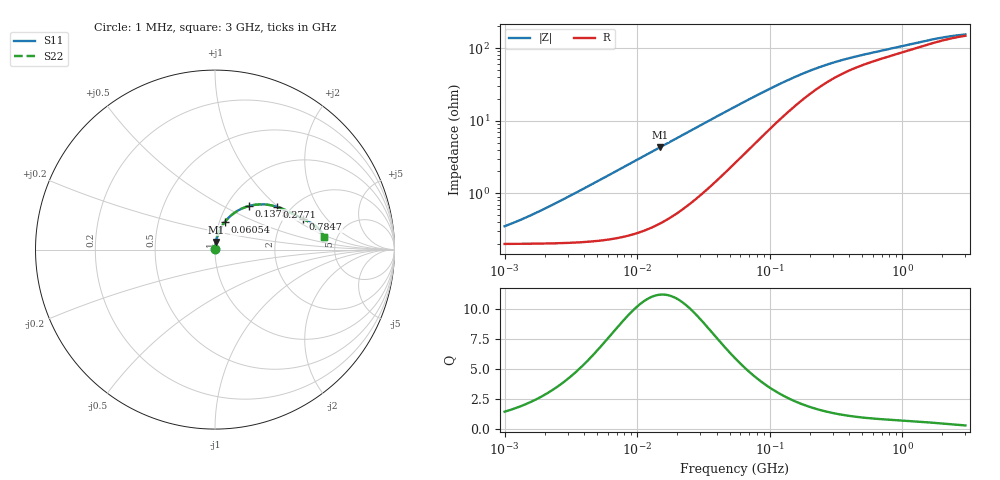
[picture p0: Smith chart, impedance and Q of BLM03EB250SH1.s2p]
! BLM03EB250SH1
# Hz S RI R 50
!Freq.(Hz) S11(Real) S11(Imag) S21(Real) S21(Imag) S12(Real) S12(Imag) S22(Real) S22(Imag)
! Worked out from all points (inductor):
!   401 points, 1 MHz to 3 GHz, reference 50 ohm
!   read as one part in series: L = 46 nH near 2.14 MHz
!   highest Q = 11.2 at 14.91 MHz (marker M1), where L = 45.9 nH
!   S11 on the Smith chart (normalised r, x): 1 MHz: 1.00, +0.01; 60.54 MHz: 1.06, +0.34; 137.5 MHz: 1.26, +0.68; 277.1 MHz: 1.70, +0.98; 784.7 MHz: 2.53, +1.19; 3 GHz: 3.96, +0.87
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1000000  0.00201 0.00288  0.998 -0.00288  0.998 -0.00288  0.00201 0.00288
1246295  0.00202 0.00359  0.998 -0.00359  0.998 -0.00359  0.00202 0.00359
1716745  0.00204 0.00494  0.998 -0.00494  0.998 -0.00494  0.00204 0.00494
2461366  0.0021 0.00708  0.9979 -0.00708  0.9979 -0.00708  0.0021 0.00708
3823119  0.00224 0.011  0.9978 -0.011  0.9978 -0.011  0.00224 0.011
8017732  0.00306 0.023  0.9969 -0.023  0.9969 -0.023  0.00306 0.023
1.461624e7  0.00551 0.0417  0.9945 -0.0417  0.9945 -0.0417  0.00551 0.0417
1.491174e7  0.00565 0.0426  0.9944 -0.0426  0.9944 -0.0426  0.00565 0.0426
2.944989e7  0.0159 0.0823  0.9841 -0.0823  0.9841 -0.0823  0.0159 0.0823
4.138676e7  0.0287 0.1125  0.9713 -0.1125  0.9713 -0.1125  0.0287 0.1125
5.477226e7  0.0468 0.1429  0.9532 -0.1429  0.9532 -0.1429  0.0468 0.1429
6.053752e7  0.0556 0.1548  0.9444 -0.1548  0.9444 -0.1548  0.0556 0.1548
9.034013e7  0.1065 0.2036  0.8935 -0.2036  0.8935 -0.2036  0.1065 0.2036
1.375402e8  0.1888 0.2428  0.8112 -0.2428  0.8112 -0.2428  0.1888 0.2428
1.680187e8  0.2349 0.251  0.7651 -0.251  0.7651 -0.251  0.2349 0.251
2.094008e8  0.2858 0.2507  0.7142 -0.2507  0.7142 -0.2507  0.2858 0.2507
2.771263e8  0.345 0.2386  0.655 -0.2386  0.655 -0.2386  0.345 0.2386
4.219165e8  0.4148 0.2094  0.5852 -0.2094  0.5852 -0.2094  0.4148 0.2094
7.846996e8  0.4908 0.1714  0.5092 -0.1714  0.5092 -0.1714  0.4908 0.1714
8.005644e8  0.4931 0.1703  0.5069 -0.1703  0.5069 -0.1703  0.4931 0.1703
1.712864e9  0.5741 0.1193  0.4259 -0.1193  0.4259 -0.1193  0.5741 0.1193
3e9  0.6089 0.0686  0.3911 -0.0686  0.3911 -0.0686  0.6089 0.0686
